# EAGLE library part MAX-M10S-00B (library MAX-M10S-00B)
GPS Modules u-blox M10 GNSS LCC module, firmware in ROM, SAW filter, LNA Source: Datasheet
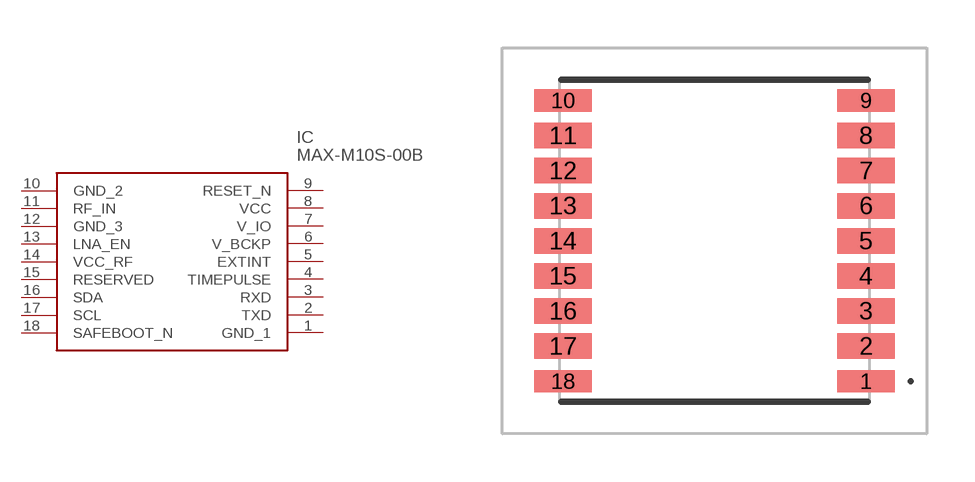
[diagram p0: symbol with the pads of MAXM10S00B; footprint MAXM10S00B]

Designator prefix IC

## MAX-M10S-00B (Arrow_Part_Number: MAX-M10S-00B; Arrow_Price-Stock: https://www.arrow.com/en/products/max-m10s-00b/u-blox?utm_currency=USD&region=nac; Description: GPS Modules u-blox M10 GNSS LCC module, firmware in ROM, SAW filter, LNA; Height: 2.7mm; Manufacturer_Name: u-blox; Manufacturer_Part_Number: MAX-M10S-00B; Mouser_Part_Number: 377-MAX-M10S-00B; Mouser_Price-Stock: https://www.mouser.co.uk/ProductDetail/u-blox/MAX-M10S-00B?qs=A6eO%252BMLsxmT0PfQYPb7LLQ%3D%3D)  [MAXM10S00B]
1  GND_1
2  TXD
3  RXD
4  TIMEPULSE
5  EXTINT
6  V_BCKP
7  V_IO
8  VCC
9  RESET_N
10  GND_2
11  RF_IN
12  GND_3
13  LNA_EN
14  VCC_RF
15  RESERVED
16  SDA
17  SCL
18  SAFEBOOT_N

## Footprint MAXM10S00B (pad centres in mm)
MAX-M10S-00B-2
smd 1.8 x 0.7: 1 4.75,-4.4; 9 4.75,4.4; 10 -4.75,4.4; 18 -4.75,-4.4
smd 1.8 x 0.8: 2 4.75,-3.3; 3 4.75,-2.2; 4 4.75,-1.1; 5 4.75,0; 6 4.75,1.1; 7 4.75,2.2; 8 4.75,3.3; 11 -4.75,3.3; 12 -4.75,2.2; 13 -4.75,1.1; 14 -4.75,0; 15 -4.75,-1.1; 16 -4.75,-2.2; 17 -4.75,-3.3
